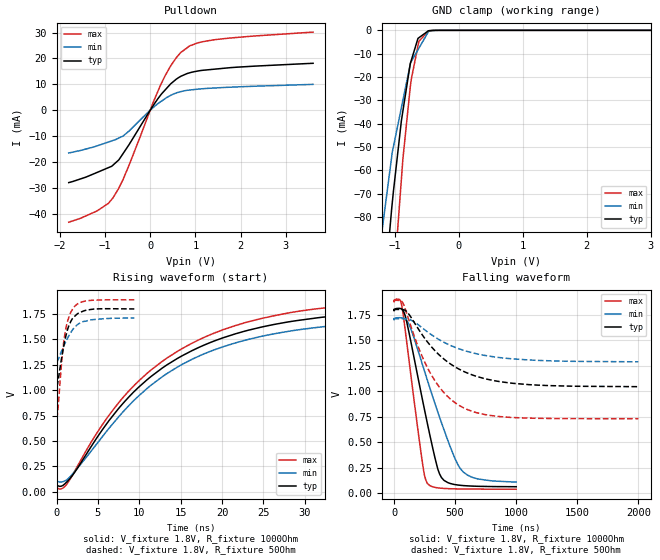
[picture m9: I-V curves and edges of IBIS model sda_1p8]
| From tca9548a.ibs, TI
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|   sda_1p8 Model
[Model]   sda_1p8
Model_type   I/O_open_drain
Polarity   Non-Inverting
Vinl  = 0.54
Vinh  =1.26
Vmeas = 0.9
Vref = 1.8
Cref = 50pF
Rref = 1000
|   typ   min   max
|   (nom PVT)   (fast PVT)   (slow PVT)
 C_comp   4.921e-12   4.514e-12   5.537e-12
[Model spec]
|subparameter
Vinl   0.54   0.513   0.567
Vinh   1.26   1.197   1.323
| Where nom  PVT is Nominal Process, 1.8V, 27C
|   Fast PVT is Strong Process,  1.89V, -40C
|   Slow PVT is Weak Process,   1.71V, 125C
[Voltage Range]   1.8   1.71   1.89
|Junction Temperature
[Temperature Range]   27   125   -40
[Pullup Reference]   1.8   1.71   1.89
[Pulldown Reference]   0   0   0
[Power Clamp Reference]   1.8   1.71   1.89
[GND Clamp Reference]   0   0   0
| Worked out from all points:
|   slope of the pulldown table from 0 to 0.27 V, typ, clamps not added: 40.4 ohm
|   GND clamp passes 1 mA (typ) near -0.51 V on its own axis
|   falling waveform, V_fixture 1.8V, R_fixture 1000Ohm: 20-80 % time 179ns typ, 270ns min, 120ns max; typ from 1.8 V to 0.064 V
|   rising waveform, V_fixture 1.8V, R_fixture 1000Ohm: 20-80 % time 14.2ns typ, 14.4ns min, 14.2ns max; typ from 0.063 V to 1.8 V
|   falling waveform, V_fixture 1.8V, R_fixture 50Ohm: 20-80 % time 389ns typ, 430ns min, 295ns max; typ from 1.8 V to 1.04 V
|   rising waveform, V_fixture 1.8V, R_fixture 50Ohm: 20-80 % time 1.19ns typ, 1.73ns min, 947ps max; typ from 1.04 V to 1.8 V
[Pulldown]
|   Voltage   I(typ)   I(min)   I(max)
-1.8V     -27.97mA   -16.54mA   -43.28mA
-1.176V   -24.06mA   -13.78mA   -38.94mA
-928mV    -22.23mA   -12.32mA   -36.06mA
-825.9mV  -21.29mA   -11.72mA   -33.96mA
-693mV    -19.19mA   -10.75mA   -30.1mA
-599.1mV  -16.74mA   -9.966mA   -26.76mA
226.8mV   5.772mA    3.238mA    9.658mA
455.5mV   10.24mA    5.765mA    17.24mA
680.4mV   13.16mA    7.204mA    22.38mA
873.2mV   14.47mA    7.81mA     24.88mA
1.382V    15.81mA    8.563mA    27.15mA
3.6V      18.15mA    9.997mA    30.21mA
[GND Clamp]
|   Voltage   I(typ)   I(min)   I(max)
-1.8V     -373.4mA   -240.8mA   -553.6mA
-1.193V   -122.1mA   -84.99mA   -189.5mA
-1.048V   -76.86mA   -54.5mA    -123mA
-1.017V   -68.5mA    -49.57mA   -109mA
-894.6mV  -38.75mA   -33.18mA   -63.83mA
-871.3mV  -34.64mA   -30.06mA   -55.22mA
-756mV    -14.32mA   -14.6mA    -24.35mA
-739mV    -12.79mA   -13.33mA   -20.84mA
-635.4mV  -3.46mA    -8.374mA   -6.626mA
-621.8mV  -3.188mA   -7.724mA   -4.761mA
-471.6mV  -181.6uA   -544.3uA   -244.9uA
3.6V      0A         0A         0A
[POWER Clamp]
|   Voltage   I(typ)   I(min)   I(max)
-1.8V     0A         0A         0A
-1.799V   0A         0A         0A
3.6V      0A         0A         0A
[Ramp]
R_load = 1000
|   typ   min   max
dV/dt_r   1.10997/1.42079e-08   0.963867/1.43583e-08   1.04197/1.41599e-08
dV/dt_f   1.04159/1.79444e-07   0.960477/2.69917e-07   1.10995/1.19571e-07
[Falling Waveform]
V_fixture = 1.8V
V_fixture_min = 1.71V
V_fixture_max = 1.89V
R_fixture = 1000Ohm
|   Time   V(typ)   V(min)   V(max)
0s        1.8V       1.71V      1.89V
64.4ns    1.803V     1.718V     1.829V
124.8ns   1.56V      1.647V     1.279V
226ns     954.2mV    1.285V     349.9mV
273.2ns   681.1mV    1.106V     95.24mV
355.2ns   249.5mV    806.1mV    53.5mV
387.6ns   154.5mV    693.2mV    49.22mV
545ns     77.55mV    237.3mV    42.12mV
681.4ns   68.43mV    141.5mV    40.72mV
999.8ns   64.02mV    109.2mV    40.09mV
[Rising Waveform]
V_fixture = 1.8V
V_fixture_min = 1.71V
V_fixture_max = 1.89V
R_fixture = 1000Ohm
|   Time   V(typ)   V(min)   V(max)
0s        63.36mV    103.5mV    40.02mV
800ps     64.96mV    100.8mV    38.9mV
1.6ns     129.2mV    145.3mV    119.4mV
6.4ns     707.5mV    631.5mV    760.5mV
11.4ns    1.134V     1.049V     1.198V
17.2ns    1.422V     1.336V     1.497V
24.6ns    1.619V     1.528V     1.703V
35ns      1.742V     1.647V     1.834V
47ns      1.793V     1.696V     1.885V
89.96ns   1.8V       1.71V      1.89V
[Falling Waveform]
V_fixture = 1.8V
V_fixture_min = 1.71V
V_fixture_max = 1.89V
R_fixture = 50Ohm
|   Time   V(typ)   V(min)   V(max)
0s        1.8V       1.71V      1.89V
73.3ns    1.799V     1.71V      1.861V
126.7ns   1.745V     1.702V     1.676V
214.7ns   1.58V      1.635V     1.383V
334.8ns   1.396V     1.53V      1.101V
447.3ns   1.278V     1.456V     938.1mV
574.7ns   1.191V     1.398V     833.4mV
744.3ns   1.122V     1.35V      770.5mV
974.7ns   1.077V     1.316V     741.7mV
2us       1.044V     1.288V     730.3mV
[Rising Waveform]
V_fixture = 1.8V
V_fixture_min = 1.71V
V_fixture_max = 1.89V
R_fixture = 50Ohm
|   Time   V(typ)   V(min)   V(max)
0s        1.043V     1.287V     730.2mV
60ps      1.043V     1.284V     734.6mV
140ps     1.07V      1.292V     784.1mV
640ps     1.331V     1.392V     1.295V
960ps     1.472V     1.45V      1.529V
1.34ns    1.599V     1.513V     1.681V
1.98ns    1.711V     1.6V       1.804V
2.78ns    1.764V     1.66V      1.861V
4.06ns    1.794V     1.691V     1.884V
9.4ns     1.8V       1.712V     1.89V
